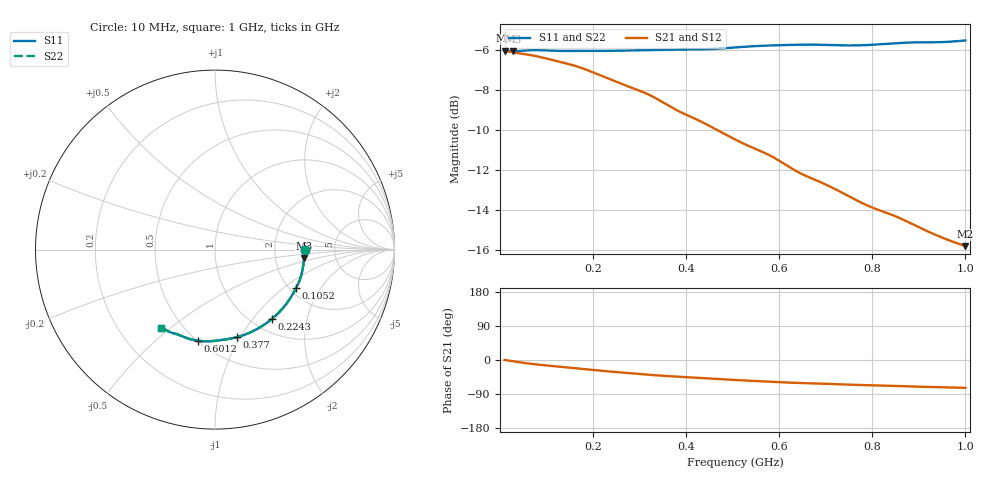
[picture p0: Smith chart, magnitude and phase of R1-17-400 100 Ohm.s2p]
!version-1
!date-02.2021
!Series
#	GHZ	S	RI	R	50.0
!	FREQ.GHZ	S11RE	S11IM	S21RE	S21IM	S12RE	S12IM	S22RE	S22IM
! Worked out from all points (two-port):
!   500 points, 10 MHz to 1 GHz, reference 50 ohm
!   highest |S21| = -6.02 dB at 10 MHz (marker M1); lowest = -15.8 dB at 1 GHz (marker M2)
!   |S21| within 3 dB of the highest: start of sweep to 381.9 MHz
!   lowest |S11| = -6.0 dB at 27.86 MHz (marker M3), VSWR 2.99, Z = 147 - j18 ohm
!   |S11| at or under -10 dB: nowhere
!   |S22| runs from -6.0 to -5.5 dB; largest |S21 - S12| = 0
!   S11 on the Smith chart (normalised r, x): 10 MHz: 3.00, -0.00; 105.2 MHz: 2.17, -1.24; 224.3 MHz: 1.21, -1.25; 377 MHz: 0.74, -0.97; 601.2 MHz: 0.50, -0.70; 1 GHz: 0.38, -0.46
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0.01  0.5 -1.56e-05  0.5 -1.86e-07  0.5 -1.86e-07  0.5 -1.56e-05
0.0278557  0.4964 -0.046  0.4945 -0.0291  0.4945 -0.0291  0.4964 -0.046
0.0655511  0.4825 -0.136  0.4805 -0.0833  0.4805 -0.0833  0.4825 -0.136
0.10523  0.4525 -0.2135  0.46 -0.1235  0.46 -0.1235  0.4525 -0.2135
0.142926  0.4147 -0.2779  0.4378 -0.1557  0.4378 -0.1557  0.4147 -0.2779
0.176653  0.376 -0.3287  0.4139 -0.1819  0.4139 -0.1819  0.376 -0.3287
0.224269  0.3158 -0.387  0.3748 -0.21  0.3748 -0.21  0.3158 -0.387
0.27982  0.2436 -0.4374  0.3333 -0.2306  0.3333 -0.2306  0.2436 -0.4374
0.315531  0.1982 -0.4608  0.3054 -0.243  0.3054 -0.243  0.1982 -0.4608
0.341323  0.166 -0.4741  0.2846 -0.2467  0.2846 -0.2467  0.166 -0.4741
0.377034  0.1231 -0.4879  0.2579 -0.246  0.2579 -0.246  0.1231 -0.4879
0.430601  0.0651 -0.4996  0.2258 -0.2448  0.2258 -0.2448  0.0651 -0.4996
0.505992  -0.011 -0.5094  0.1809 -0.2388  0.1809 -0.2388  -0.011 -0.5094
0.551623  -0.0531 -0.5108  0.1597 -0.2338  0.1597 -0.2338  -0.0531 -0.5108
0.601222  -0.0944 -0.5074  0.1378 -0.226  0.1378 -0.226  -0.0944 -0.5074
0.636934  -0.1227 -0.5026  0.1234 -0.2172  0.1234 -0.2172  -0.1227 -0.5026
0.670661  -0.1471 -0.4964  0.114 -0.2106  0.114 -0.2106  -0.1471 -0.4964
0.728196  -0.182 -0.4825  0.0971 -0.2006  0.0971 -0.2006  -0.182 -0.4825
0.787715  -0.2094 -0.4721  0.0829 -0.188  0.0829 -0.188  -0.2094 -0.4721
0.835331  -0.233 -0.4657  0.0744 -0.181  0.0744 -0.181  -0.233 -0.4657
0.90477  -0.2657 -0.4525  0.0597 -0.1696  0.0597 -0.1696  -0.2657 -0.4525
1  -0.3015 -0.4363  0.046 -0.1556  0.046 -0.1556  -0.3015 -0.4363
